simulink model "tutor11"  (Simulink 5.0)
settings: Solver=ode45  SolverMode=SingleTasking  StartTime=0.0  StopTime=10  RelTol=1e-3  AbsTol=1e-3
libraries: simulink x1

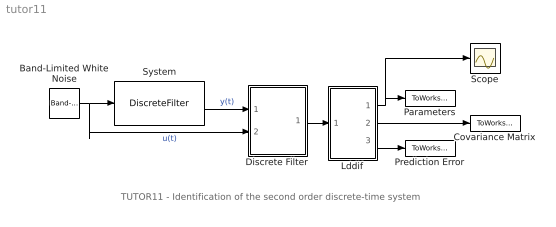
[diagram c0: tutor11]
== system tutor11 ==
  note: TUTOR11 - Identification of the second order discrete-time system
  Band-Limited White Noise : simulink/Sources/Band-Limited White Noise  Cov=[0.1]  Ts=0.1  seed=[23341]
  Covariance Matrix : ToWorkspace  VariableName=CovMatrix  SaveFormat=Array
  Discrete Filter : Subsystem  mask(D-Filter){par=[1,1], cit=[2], men=[2], ts=[1], Ds=[0]}
      mask prompts: par "No. of inputs and outputs -  [in,out]:"; cit "Numerator degree -  [dn]:"; men "Denominator degree -  [dd]:"; ts "Sampling time - [ts]:"; Ds "Discrete time delay - [D]:"
      mask help: D-filter: Discrete filter Authors: Lubos Cirka and Miroslav Fikar 1998 - 2006
      mask init:
      | % State-space realisation of discete-time MIMO filters
      | %
      | % Input:
      | %    y1(k), ..., yn(k), u1(k), ..., um(k)
      | % Output:
      | %    y(k), y(k-1), y(k-2) ..., u(k-1-Ds), ...
      | 
      | % State-space realisation of the output filter
      | 
      | in=par(1); out=par(2);
      | A0=zeros(men*out);
      | A0(out+1:men*out,1:(men-1)*out)=eye((men-1)*out);
      | Ay=A0;
      | 
      | B0=-eye(out);
      | B1=zeros((men-1)*out,out);
      | By=[B0;B1];
      | 
      | C0=zeros(out,men*out);
      | C1=eye(men*out);
      | Cy=[C0;C1];
      | 
      | D1=eye(out);
      | D2=zeros(men*out,out);
      | Dy=[D1;D2];
      | 
      | % State-space realisation of the input filter
      | 
      | a0=zeros(in,(cit+Ds)*in);
      | a1=eye((cit+Ds-1)*in);
      | a2=zeros((cit+Ds-1)*in,in);
      | Au=[a0;[a1 a2]];
      | 
      | b0=eye(in);
      | b1=zeros((cit+Ds-1)*in,in);
      | Bu=[b0;b1];
      | 
      | c0=zeros(cit*in,Ds*in);
      | c1=eye(cit*in);
      | Cu=[c0 c1];
      | 
      | Du=zeros(cit*in,in);
  Lddif : Subsystem  mask(LDDIF){par=[4,1], L=[0.985], d=[0.01], poc=[0 0 0 0], kov=[10e6], ts=[1]}
      mask prompts: par "No. of estimated parameters and outputs - [n,m]:"; L "Exponential forgetting - [L]:"; d "Bittanti's correction - [d]:"; poc "Initial parameter estimates - [theta(1) ... theta(n)]:"; kov "Covariance matrix (see help, standard - [10e6]):"; ts "Sampling period - [ts]:"
      mask help: LDDIF: + Bittanti's corrections Authors: Lubos Cirka and Miroslav Fikar 1998 - 2006
      mask init:
      | n=par(1); m=par(2);
  Parameters : ToWorkspace  VariableName=BA  SaveFormat=Array
  Prediction Error : ToWorkspace  VariableName=PredError  SaveFormat=Array
  Scope : Scope
  System : DiscreteFilter  Numerator=[0 0.8 0.2]  Denominator=[1 -0.5 0.06]
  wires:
  System/1 -> Discrete Filter/1(y)  "y(t)"
  Band-Limited White Noise/1 -> System/1, Discrete Filter/2(u)  "u(t)"
  Discrete Filter/1("y, z") -> Lddif/1("y, z")
  Lddif/2(covariance matrix) -> Covariance Matrix/1
  Lddif/3(prediction error) -> Prediction Error/1
  Lddif/1(theta) -> Parameters/1, Scope/1

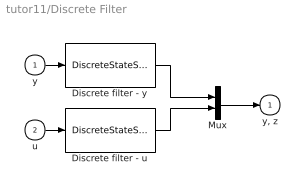
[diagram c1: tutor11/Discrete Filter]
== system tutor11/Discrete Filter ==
  y : Inport
  u : Inport  Port=2
  Discrete filter - u : DiscreteStateSpace  A=Au  B=Bu  C=Cu  D=Du  SampleTime=ts
  Discrete filter - y : DiscreteStateSpace  A=Ay  B=By  C=Cy  D=Dy  SampleTime=ts
  Mux : Mux  Inputs=2
  "y, z" : Outport  InitialOutput=0
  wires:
  y/1 -> Discrete filter - y/1
  u/1 -> Discrete filter - u/1
  Discrete filter - y/1 -> Mux/1
  Discrete filter - u/1 -> Mux/2
  Mux/1 -> "y, z"/1

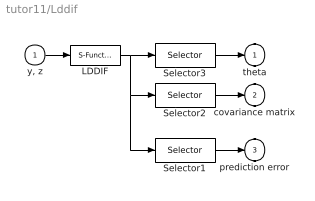
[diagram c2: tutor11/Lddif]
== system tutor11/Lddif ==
  "y, z" : Inport
  LDDIF : S-Function  FunctionName=lddif_s  Parameters=m, n, L, d, poc, kov, ts
  Selector1 : Selector  Elements=[n*m+n*n+1:1:n*m+n*n+m]  InputPortWidth=n*m+n*n+m
  Selector2 : Selector  Elements=[n*m+1:1:n*m+n*n]  InputPortWidth=n*m+n*n+m
  Selector3 : Selector  Elements=[1:1:n*m]  InputPortWidth=n*m+n*n+m
  theta : Outport  InitialOutput=0
  covariance matrix : Outport  Port=2  InitialOutput=0
  prediction error : Outport  Port=3  InitialOutput=0
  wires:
  "y, z"/1 -> LDDIF/1
  LDDIF/1 -> Selector1/1, Selector2/1, Selector3/1
  Selector2/1 -> covariance matrix/1
  Selector3/1 -> theta/1
  Selector1/1 -> prediction error/1
